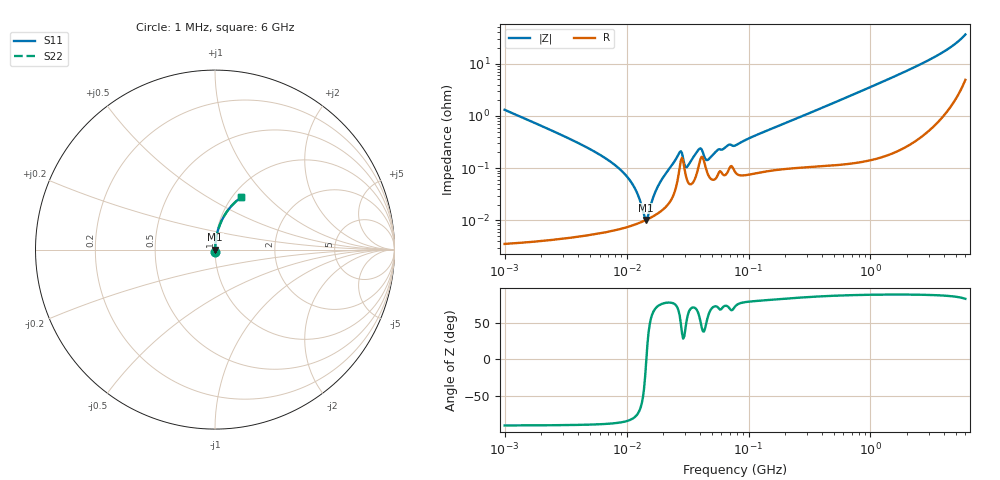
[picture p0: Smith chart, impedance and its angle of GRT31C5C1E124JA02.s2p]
!Murata Part Number: GRT31C5C1E124JA02
!These Parameters are Measured in Series Mode Connection
!Data Generated on Jun 19, 2026
!  o--ll--o
!Port1  Port2
!  o------o
!Operation Temp=25[degC], DC Bias Voltage=0[V]
!Freq. Start=1000[kHz] Stop=6[GHz] 401[Steps]
# Hz S RI R 50
!Freq.(Hz) S11(Real) S11(Imag) S21(Real) S21(Imag) S12(Real) S12(Imag) S22(Real) S22(Imag)
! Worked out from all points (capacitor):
!   401 points, 1 MHz to 6 GHz, reference 50 ohm
!   read as one part in series: C = 121 nF near 1.044 MHz
!   lowest |Z| = 10.2 mohm at 14.51 MHz (marker M1)
!   series resonance near 14.53 MHz, so ESL is about 990 pH
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1000000  0.000208 -0.0131  0.9998 0.0131  0.9998 0.0131  0.000208 -0.0131
4293785  5.78e-05 -0.0028  0.9999 0.0028  0.9999 0.0028  5.78e-05 -0.0028
7080828  6.27e-05 -0.00143  0.9999 0.00143  0.9999 0.00143  6.27e-05 -0.00143
9812162  7.35e-05 -0.000739  0.9999 0.000739  0.9999 0.000739  7.35e-05 -0.000739
1.193364e7  8.48e-05 -0.000367  0.9999 0.000367  0.9999 0.000367  8.48e-05 -0.000367
1.389603e7  9.78e-05 -8.3e-05  0.9999 8.3e-05  0.9999 8.3e-05  9.78e-05 -8.3e-05
1.451381e7  0.000102 -1.5e-06  0.9999 1.5e-06  0.9999 1.5e-06  0.000102 -1.5e-06
1.515906e7  0.000108 8.08e-05  0.9999 -8.08e-05  0.9999 -8.08e-05  0.000108 8.08e-05
1.690048e7  0.000124 0.000292  0.9999 -0.000292  0.9999 -0.000292  0.000124 0.000292
1.843659e7  0.000141 0.000471  0.9999 -0.000471  0.9999 -0.000471  0.000141 0.000471
2.727078e7  0.00104 0.00174  0.999 -0.00174  0.999 -0.00174  0.00104 0.00174
2.848316e7  0.00158 0.00113  0.9984 -0.00113  0.9984 -0.00113  0.00158 0.00113
3.107204e7  0.00063 0.000823  0.9994 -0.000823  0.9994 -0.000823  0.00063 0.000823
3.947016e7  0.00123 0.00199  0.9988 -0.00199  0.9988 -0.00199  0.00123 0.00199
4.596069e7  0.000814 0.00117  0.9992 -0.00117  0.9992 -0.00117  0.000814 0.00117
5.589783e7  0.000739 0.00212  0.9993 -0.00212  0.9993 -0.00212  0.000739 0.00212
6.947823e7  0.000987 0.00265  0.999 -0.00265  0.999 -0.00265  0.000987 0.00265
7.745967e7  0.000859 0.00256  0.9991 -0.00256  0.9991 -0.00256  0.000859 0.00256
3.325952e8  0.0012 0.0119  0.9988 -0.0119  0.9988 -0.0119  0.0012 0.0119
1.428092e9  0.00446 0.0513  0.9955 -0.0513  0.9955 -0.0513  0.00446 0.0513
3.883682e9  0.0347 0.1565  0.9653 -0.1565  0.9653 -0.1565  0.0347 0.1565
6e9  0.1472 0.2925  0.8528 -0.2925  0.8528 -0.2925  0.1472 0.2925
